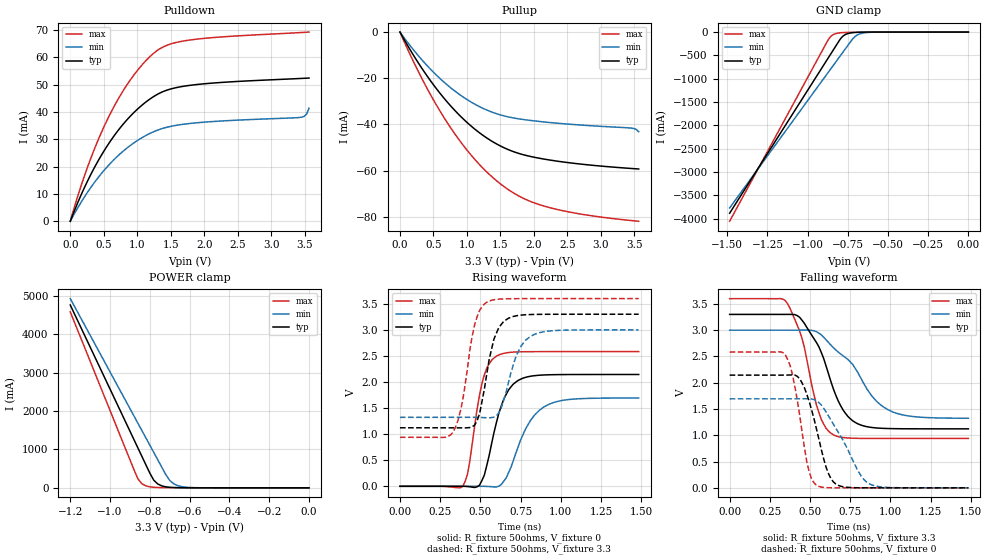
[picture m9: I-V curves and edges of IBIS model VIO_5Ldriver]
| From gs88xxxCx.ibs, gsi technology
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|  signals   DQA1-DQA9, DQB1-DQB9, DQC1-DQC9, DQD1-DQD9
[Model]   VIO_5Ldriver
Model_type   I/O
Polarity   Non-Inverting
Vinl  =   0.75v
Vinh  =   1.75v
Vmeas =   0.90v
Cref  =   0pF
Rref  =   50
Vref  =   0.90v
|  variable   typ   min   max
C_comp   3.0pF   2.5pF   3.5pF
|  variable   typ   min   max
[Temperature Range]   50   0   100
|  variable   typ   min   max
[Voltage Range]   3.3   3.0   3.6
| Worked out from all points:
|   slope of the pulldown table from 0 to 0.495 V, typ, clamps not added: 19.5 ohm
|   slope of the pullup table from 0 to 0.495 V, typ, clamps not added: 21.9 ohm
|   GND clamp passes 1 mA (typ) near -0.61 V on its own axis
|   POWER clamp passes 1 mA (typ) near -0.59 V on its own axis
|   rising waveform, R_fixture 50ohms, V_fixture 0: 20-80 % time 111ps typ, 148ps min, 82.3ps max; typ from 0 V to 2.14 V
|   rising waveform, R_fixture 50ohms, V_fixture 3.3: 20-80 % time 84.4ps typ, 103ps min, 84.7ps max; typ from 1.12 V to 3.3 V
|   falling waveform, R_fixture 50ohms, V_fixture 3.3: 20-80 % time 172ps typ, 264ps min, 127ps max; typ from 3.3 V to 1.12 V
|   falling waveform, R_fixture 50ohms, V_fixture 0: 20-80 % time 109ps typ, 178ps min, 82.4ps max; typ from 2.14 V to 0 V
[Pulldown]
| voltage   typ   min   max
0V        -445.6pA   -1.181nA   -285.9pA
144mV     8.659mA    6.25mA     11.68mA
288mV     16.23mA    11.72mA    21.85mA
576mV     28.52mA    20.62mA    38.35mA
900mV     38.58mA    27.83mA    51.88mA
1.08V     42.72mA    30.74mA    57.51mA
1.26V     45.91mA    32.95mA    61.84mA
1.476V    48.28mA    34.64mA    64.76mA
1.8V      49.83mA    35.86mA    66.44mA
3.456V    52.32mA    38.14mA    69.14mA
3.528V    52.41mA    39.22mA    69.25mA
3.564V    52.46mA    41.4mA     69.31mA
[Pullup]
| voltage (VDDQ-Vout)   typ   min   max
0V        394.9pA    1.311nA    168.6pA
180mV     -8.998mA   -6.92mA    -11.49mA
360mV     -17.1mA    -13.09mA   -21.93mA
720mV     -30.75mA   -23.23mA   -39.81mA
1.08V     -41.11mA   -30.6mA    -53.87mA
1.26V     -45.12mA   -33.28mA   -59.52mA
1.476V    -48.95mA   -35.65mA   -65.16mA
1.8V      -52.75mA   -37.68mA   -71.34mA
2.196V    -55.2mA    -39.04mA   -75.67mA
2.736V    -57.25mA   -40.31mA   -78.95mA
3.456V    -59.05mA   -41.57mA   -81.58mA
3.564V    -59.27mA   -43.17mA   -81.89mA
[GND Clamp]
| voltage   typ   min   max
-1.485V   -3.884A    -3.771A    -4.056A
-885mV    -626.9mA   -926.9mA   -247.2mA
-870mV    -545.6mA   -856mA     -153.5mA
-855mV    -464.4mA   -785mA     -89.11mA
-825mV    -301.9mA   -643.2mA   -32.88mA
-795mV    -141.5mA   -501.4mA   -15.38mA
-780mV    -86.61mA   -430.5mA   -11.65mA
-750mV    -32.85mA   -288.8mA   -7.734mA
-705mV    -8.727mA   -95.28mA   -4.834mA
-660mV    -2.907mA   -24.97mA   -2.925mA
-555mV    -316.7uA   -1.176mA   -484.9uA
0V        -445.6pA   -1.181nA   -285.9pA
[POWER Clamp]
| voltage (VDDQ-Vout)   typ   min   max
-1.2V     4.765A     4.931A     4.585A
-880mV    1.258A     1.875A     474.1mA
-860mV    1.039A     1.684A     234.3mA
-840mV    820.4mA    1.493A     107.4mA
-820mV    601.5mA    1.302A     50.64mA
-780mV    197.3mA    920.5mA    14.28mA
-760mV    99.71mA    729.7mA    9.034mA
-720mV    26.23mA    348.2mA    4.898mA
-700mV    13.96mA    192.6mA    3.916mA
-660mV    4.495mA    57.55mA    2.579mA
-560mV    510.5uA    2.941mA    648.3uA
0V        395pA      1.311nA    168.9pA
[Ramp]
| voltage   typ   min   max
dV/dt_r   0.46/174p   0.27/249p   0.72/134p
dV/dt_f   0.47/106p   0.32/123p   0.64/90p
R_load  =   50ohms
[Rising Waveform]
C_fixture =   0.0pF
R_fixture =   50ohms
V_fixture =   0
| Time   V(typ)   V(min)   V(max)
0s        5.291nV    17.82nV    2.677nV
390ps     65.54uV    312.3uV    -2.05mV
420ps     -4.733mV   544.3uV    230mV
495ps     20.83mV    393.9uV    1.748V
540ps     397.8mV    -2.623mV   2.264V
600ps     1.222V     -11.48mV   2.496V
705ps     1.96V      492.5mV    2.574V
795ps     2.101V     1.173V     2.582V
900ps     2.136V     1.531V     2.583V
1.485ns   2.144V     1.693V     2.583V
[Rising Waveform]
C_fixture =   0.0pF
R_fixture =   50ohms
V_fixture =   3.3
V_fixture_min =  3.0
V_fixture_max =  3.6
| Time   V(typ)   V(min)   V(max)
0s        1.122V     1.323V     939.2mV
330ps     1.121V     1.323V     1.034V
390ps     1.12V      1.323V     1.644V
465ps     1.175V     1.323V     3.102V
495ps     1.389V     1.321V     3.37V
540ps     2.153V     1.315V     3.529V
615ps     3.043V     1.41V      3.59V
720ps     3.268V     2.475V     3.599V
810ps     3.294V     2.872V     3.6V
1.485ns   3.3V       3V         3.6V
[Falling Waveform]
C_fixture =   0.0pF
R_fixture =   50ohms
V_fixture =   3.3
V_fixture_min =  3.0
V_fixture_max =  3.6
| Time   V(typ)   V(min)   V(max)
0s        3.3V       3V         3.6V
345ps     3.3V       3V         3.567V
465ps     3.129V     3.001V     2.673V
555ps     2.685V     2.945V     1.433V
645ps     1.885V     2.668V     1.011V
705ps     1.485V     2.514V     957.8mV
765ps     1.277V     2.35V      944.3mV
885ps     1.148V     1.746V     939.8mV
975ps     1.129V     1.503V     939.5mV
1.485ns   1.123V     1.324V     939.3mV
[Falling Waveform]
C_fixture =   0.0pF
R_fixture =   50ohms
V_fixture =   0
| Time   V(typ)   V(min)   V(max)
0s        2.144V     1.693V     2.583V
345ps     2.145V     1.693V     2.543V
390ps     2.148V     1.693V     2.163V
435ps     2.08V      1.694V     1.392V
480ps     1.78V      1.696V     494.3mV
540ps     1.121V     1.658V     47.73mV
600ps     391.1mV    1.443V     4.465mV
645ps     114.3mV    1.212V     836.3uV
855ps     412.3uV    100.3mV    10.3uV
1.485ns   1.082uV    4.087uV    454.6nV
